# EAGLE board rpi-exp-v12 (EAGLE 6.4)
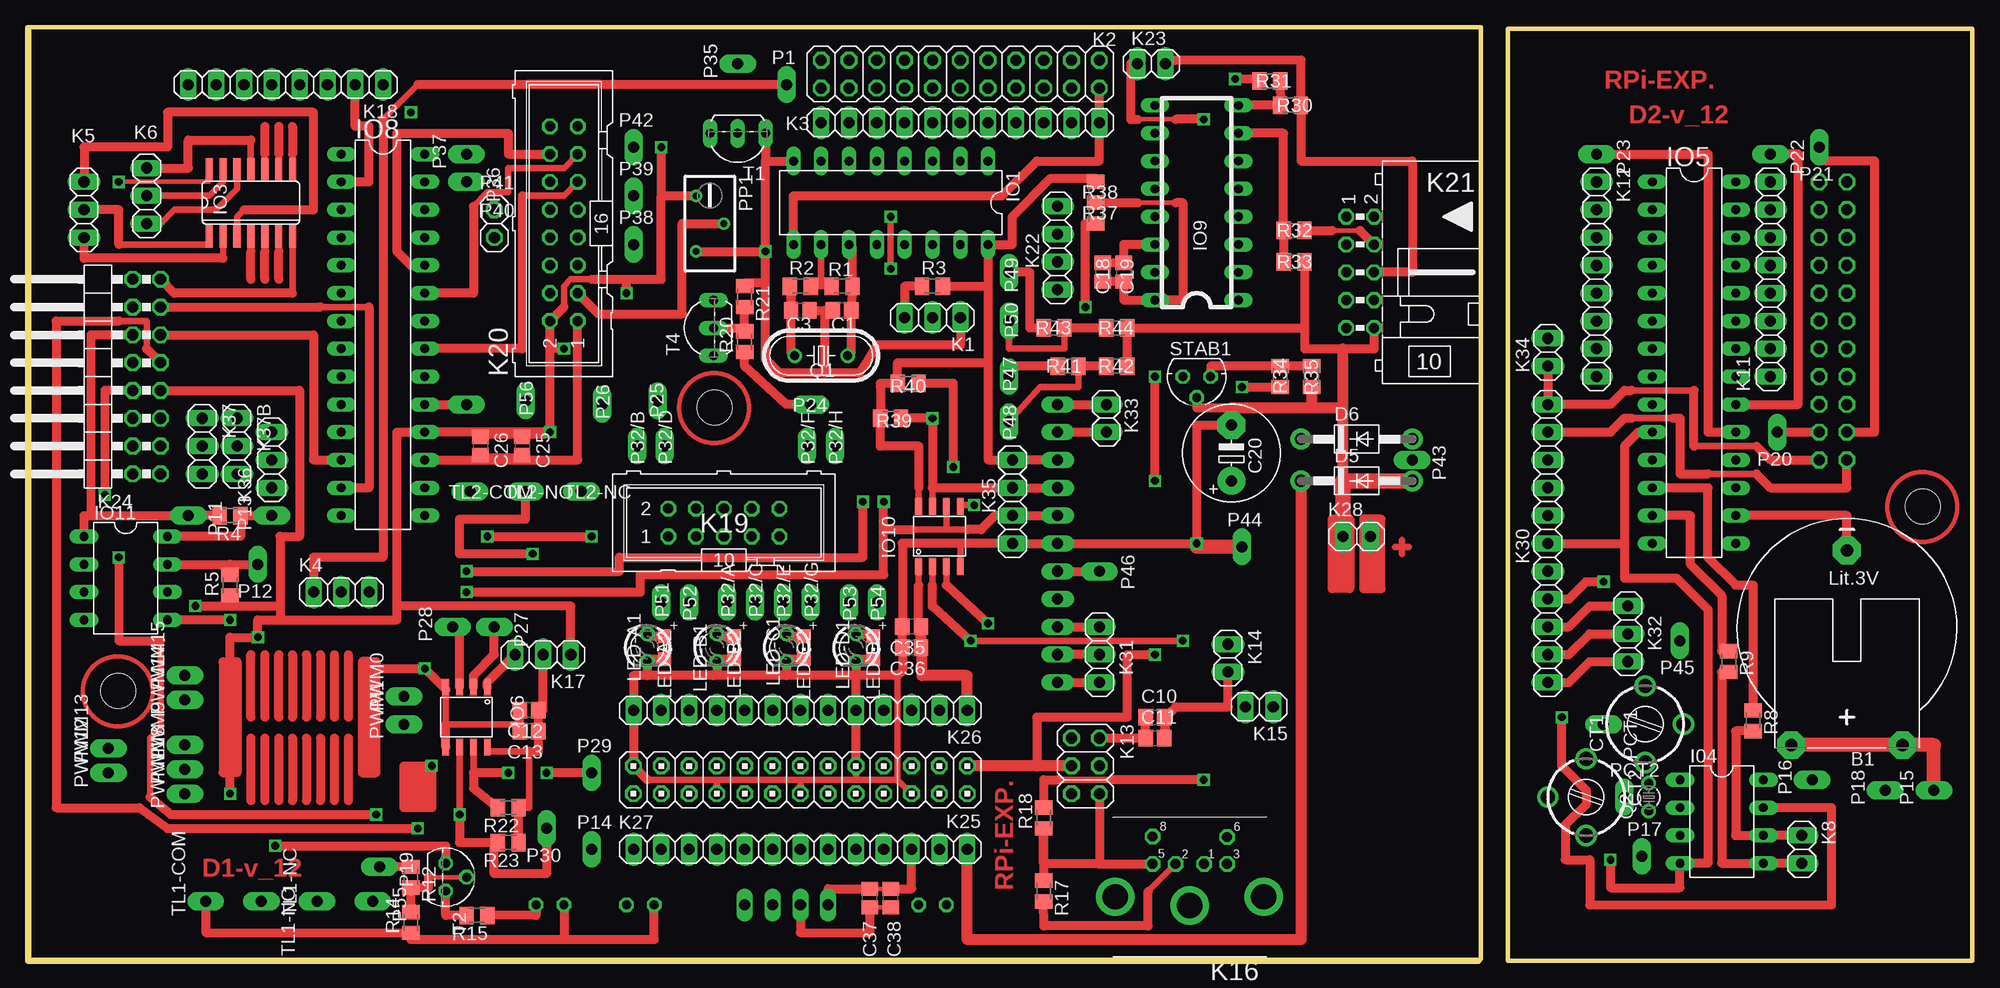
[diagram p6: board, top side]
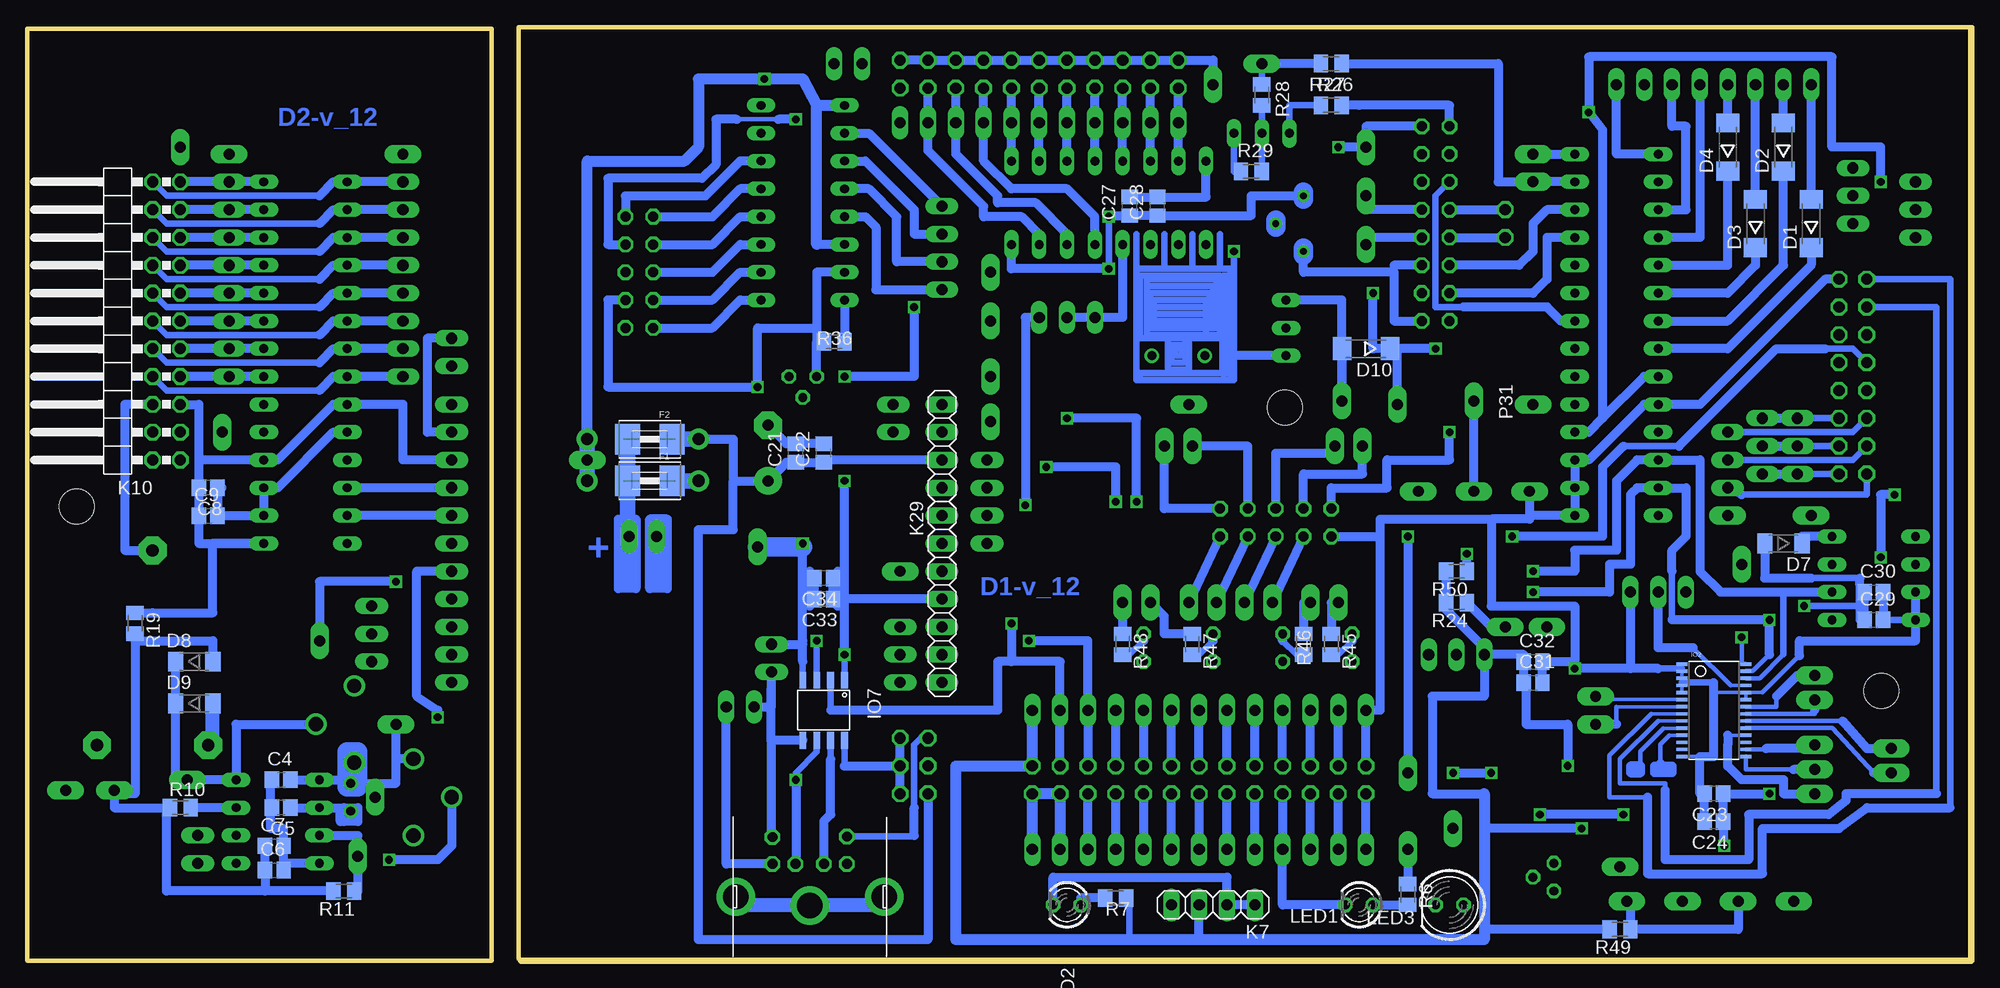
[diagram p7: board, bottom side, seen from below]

Size 177.57 x 85.23 mm. Coordinates in mm from the lower left corner, seen from the top.
Outline: 132.7,0.15 132.7,85.23 0,85.23 0,0.47
Outline: 132.49,0 0.09,0 0.09,85.09
Outline: 135.18,85.09 177.57,85.09 177.57,0 135.18,0 135.18,85.09
Copper layers (1*16): Top 0.035mm / dielectric 1.5mm / Bottom 0.035mm
Design rules "default": minimum track width 10mil, minimum drill 24mil, track to track 8mil, track to pad 8mil, pad to pad 8mil, via to via 8mil, smd to smd 8mil, copper to edge 40mil, drill to drill 8mil, minimum pad ring 10mil, minimum via ring 8mil, stop-mask expansion 4mil, vias tented up to drill 0mil, thermal gap 10mil
Holes 3.2 mm at 62.76,50.5 8.3,24.63 173.08,41.46

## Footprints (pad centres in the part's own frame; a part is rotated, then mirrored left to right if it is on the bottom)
CR2032H = drill 1.118 pad 2.54 octagon: + 5.08,10.795; +@1 -5.08,10.795; - 0,-6.985
0805 = smd 1.3 x 1.5: 1 -0.85,0; 2 0.85,0
E5-8,5 = drill 1.016 pad 2.54: + -2.54,0 | drill 1.016 pad 2.54 octagon: - 2.54,0
CTRIM3040.427 = drill 1.3: 1A -3.5,0; 1B 3.5,0; 2 0,-3.5
SOD106A-R = smd 1.7 x 2.1: A 2.2,0; C -2.2,0
DO41-10 = drill 1.118 pad 1.93: A 5.08,0; C -5.08,0
SOD80 = smd 1.4 x 1.8: 1 -1.7,0; 2 1.7,0
1812 = smd 2.286 x 2.794: 1 -2.046,0; 2 2.046,0
DIL08 = drill 0.813 long: 1 -3.81,-3.81; 2 -1.27,-3.81; 3 1.27,-3.81; 4 3.81,-3.81; 5 3.81,3.81; 6 1.27,3.81; 7 -1.27,3.81; 8 -3.81,3.81
DIL16 = drill 0.813 long: 1 -8.89,-3.81; 2 -6.35,-3.81; 3 -3.81,-3.81; 4 -1.27,-3.81; 5 1.27,-3.81; 6 3.81,-3.81; 7 6.35,-3.81; 8 8.89,-3.81; 9 8.89,3.81; 10 6.35,3.81; 11 3.81,3.81; 12 1.27,3.81; 13 -1.27,3.81; 14 -3.81,3.81; 15 -6.35,3.81; 16 -8.89,3.81
TSSOP28 = smd 0.305 x 0.991: 1 -4.225,-2.918; 2 -3.575,-2.918; 3 -2.925,-2.918; 4 -2.275,-2.918; 5 -1.625,-2.918; 6 -0.975,-2.918; 7 -0.325,-2.918; 8 0.325,-2.918; 9 0.975,-2.918; 10 1.625,-2.918; 11 2.275,-2.918; 12 2.925,-2.918; 13 3.575,-2.918; 14 4.225,-2.918; 15 4.225,2.918; 16 3.575,2.918; 17 2.925,2.918; 18 2.275,2.918; 19 1.625,2.918; 20 0.975,2.918; 21 0.325,2.918; 22 -0.325,2.918; 23 -0.975,2.918; 24 -1.625,2.918; 25 -2.275,2.918; 26 -2.925,2.918; 27 -3.575,2.918; 28 -4.225,2.918
SO14 = smd 0.66 x 2.032: 1 -3.81,-3.073; 2 -2.54,-3.073; 3 -1.27,-3.073; 4 0,-3.073; 5 1.27,-3.073; 6 2.54,-3.073; 7 3.81,-3.073; 8 3.81,3.073; 9 2.54,3.073; 10 1.27,3.073; 11 0,3.073; 12 -1.27,3.073; 13 -2.54,3.073; 14 -3.81,3.073
DIL28-3 = drill 0.813 long: 1 -16.51,-3.81; 2 -13.97,-3.81; 3 -11.43,-3.81; 4 -8.89,-3.81; 5 -6.35,-3.81; 6 -3.81,-3.81; 7 -1.27,-3.81; 8 1.27,-3.81; 9 3.81,-3.81; 10 6.35,-3.81; 11 8.89,-3.81; 12 11.43,-3.81; 13 13.97,-3.81; 14 16.51,-3.81; 15 16.51,3.81; 16 13.97,3.81; 17 11.43,3.81; 18 8.89,3.81; 19 6.35,3.81; 20 3.81,3.81; 21 1.27,3.81; 22 -1.27,3.81; 23 -3.81,3.81; 24 -6.35,3.81; 25 -8.89,3.81; 26 -11.43,3.81; 27 -13.97,3.81; 28 -16.51,3.81
SO8-COOL = smd 0.61 x 1.524: 1 -1.905,-2.743; 2 -0.635,-2.743; 3 0.635,-2.743; 4 1.905,-2.743; 5 1.905,2.743; 6 0.635,2.743; 7 -0.635,2.743; 8 -1.905,2.743
DIP16 = drill 0.8 long: P$1 -10.16,-3.81; P$2 -7.62,-3.81; P$3 -5.08,-3.81; P$4 -2.54,-3.81; P$5 0,-3.81; P$6 2.54,-3.81; P$7 5.08,-3.81; P$8 7.62,-3.81; P$9 7.62,3.81; P$10 5.08,3.81; P$11 2.54,3.81; P$12 0,3.81; P$13 -2.54,3.81; P$14 -5.08,3.81; P$15 -7.62,3.81; P$16 -10.16,3.81
1X03 = drill 1.016 long: 1 -2.54,0; 2 0,0; 3 2.54,0
2X11 = drill 1.016 octagon: 1 -12.7,-1.27; 2 -12.7,1.27; 3 -10.16,-1.27; 4 -10.16,1.27; 5 -7.62,-1.27; 6 -7.62,1.27; 7 -5.08,-1.27; 8 -5.08,1.27; 9 -2.54,-1.27; 10 -2.54,1.27; 11 0,-1.27; 12 0,1.27; 13 2.54,-1.27; 14 2.54,1.27; 15 5.08,-1.27; 16 5.08,1.27; 17 7.62,-1.27; 18 7.62,1.27; 19 10.16,-1.27; 20 10.16,1.27; 21 12.7,-1.27; 22 12.7,1.27
1X11 = drill 1.016 long: 1 -12.7,0; 2 -10.16,0; 3 -7.62,0; 4 -5.08,0; 5 -2.54,0; 6 0,0; 7 2.54,0; 8 5.08,0; 9 7.62,0; 10 10.16,0; 11 12.7,0
1X04 = drill 1.016 long: 1 -3.81,0; 2 -1.27,0; 3 1.27,0; 4 3.81,0
1X02 = drill 1.016 long: 1 -1.27,0; 2 1.27,0
2X11/90 = drill 1.016 octagon: 1 -12.7,-6.35; 2 -12.7,-3.81; 3 -10.16,-6.35; 4 -10.16,-3.81; 5 -7.62,-6.35; 6 -7.62,-3.81; 7 -5.08,-6.35; 8 -5.08,-3.81; 9 -2.54,-6.35; 10 -2.54,-3.81; 11 0,-6.35; 12 0,-3.81; 13 2.54,-6.35; 14 2.54,-3.81; 15 5.08,-6.35; 16 5.08,-3.81; 17 7.62,-6.35; 18 7.62,-3.81; 19 10.16,-6.35; 20 10.16,-3.81; 21 12.7,-6.35; 22 12.7,-3.81
1X08 = drill 1.016 long: 1 -8.89,0; 2 -6.35,0; 3 -3.81,0; 4 -1.27,0; 5 1.27,0; 6 3.81,0; 7 6.35,0; 8 8.89,0
2X03 = drill 1.016 octagon: 1 -2.54,-1.27; 2 -2.54,1.27; 3 0,-1.27; 4 0,1.27; 5 2.54,-1.27; 6 2.54,1.27
M_DIN6 = drill 0.9 pad 1.422 octagon: 1 -1.3,-3.75; 2 1.3,-3.75; 3 -3.4,-3.75; 5 3.4,-3.75; 6 -3.4,-6.2; 8 3.4,-6.25 | drill 2.3 pad 3.5: SH1 6.8,-0.75; SH2 0,0.05; SH3 -6.75,-0.75
ML10 = drill 0.914 octagon: 1 -5.08,-1.27; 2 -5.08,1.27; 3 -2.54,-1.27; 4 -2.54,1.27; 5 0,-1.27; 6 0,1.27; 7 2.54,-1.27; 8 2.54,1.27; 9 5.08,-1.27; 10 5.08,1.27
ML16 = drill 0.914 octagon: 1 -8.89,-1.27; 2 -8.89,1.27; 3 -6.35,-1.27; 4 -6.35,1.27; 5 -3.81,-1.27; 6 -3.81,1.27; 7 -1.27,-1.27; 8 -1.27,1.27; 9 1.27,-1.27; 10 1.27,1.27; 11 3.81,-1.27; 12 3.81,1.27; 13 6.35,-1.27; 14 6.35,1.27; 15 8.89,-1.27; 16 8.89,1.27
ML10L = drill 0.914 octagon: 1 -5.08,-1.27; 2 -5.08,1.27; 3 -2.54,-1.27; 4 -2.54,1.27; 5 0,-1.27; 6 0,1.27; 7 2.54,-1.27; 8 2.54,1.27; 9 5.08,-1.27; 10 5.08,1.27
2X08/90 = drill 1.016 octagon: 1 -8.89,-6.35; 2 -8.89,-3.81; 3 -6.35,-6.35; 4 -6.35,-3.81; 5 -3.81,-6.35; 6 -3.81,-3.81; 7 -1.27,-6.35; 8 -1.27,-3.81; 9 1.27,-6.35; 10 1.27,-3.81; 11 3.81,-6.35; 12 3.81,-3.81; 13 6.35,-6.35; 14 6.35,-3.81; 15 8.89,-6.35; 16 8.89,-3.81
2X13 = drill 1.016 octagon: 1 -15.24,-1.27; 2 -15.24,1.27; 3 -12.7,-1.27; 4 -12.7,1.27; 5 -10.16,-1.27; 6 -10.16,1.27; 7 -7.62,-1.27; 8 -7.62,1.27; 9 -5.08,-1.27; 10 -5.08,1.27; 11 -2.54,-1.27; 12 -2.54,1.27; 13 0,-1.27; 14 0,1.27; 15 2.54,-1.27; 16 2.54,1.27; 17 5.08,-1.27; 18 5.08,1.27; 19 7.62,-1.27; 20 7.62,1.27; 21 10.16,-1.27; 22 10.16,1.27; 23 12.7,-1.27; 24 12.7,1.27; 25 15.24,-1.27; 26 15.24,1.27
1X13 = drill 1.016 long: 1 -15.24,0; 2 -12.7,0; 3 -10.16,0; 4 -7.62,0; 5 -5.08,0; 6 -2.54,0; 7 0,0; 8 2.54,0; 9 5.08,0; 10 7.62,0; 11 10.16,0; 12 12.7,0; 13 15.24,0
LED3MM = drill 0.813 octagon: A -1.27,0; K 1.27,0
LED5MM = drill 0.813 octagon: A -1.27,0; K 1.27,0
CHIP-LED0805 = smd 1.2 x 1.2: A 0,-1.05; C 0,1.05
1X01_OVAL = drill 1 pad 1.676 long: 1 0,0
1X01 = drill 1.016 octagon: 1 0,0
RTRIM3296Y = drill 0.61: 1 1.27,-2.54; 2 -1.27,0; 3 1.27,2.54
HC49U-V = drill 0.813: 1 -2.413,0; 2 2.413,0
TC26V = drill 0.813: 1 -1.27,0; 2 1.27,0
M0805 = smd 1.3 x 1.6: 1 -0.95,0; 2 0.95,0
TO92 = drill 0.813 octagon: 1 -1.27,0; 2 0,1.905; 3 1.27,0
TO92-EBC-OVAL = drill 0.813 long: B 0,-1.27; C 2.54,-1.27; E -2.54,-1.27
TO92' = drill 0.813 octagon: 1 1.27,0; 2 0,1.905; 3 -1.27,0

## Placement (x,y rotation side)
B1  CR2032H  [CR2032H]  166.14,30.48 180 top
C1  22p - 37p  [0805]  74.39,59.37 180 top
C3  100p  [0805]  70.58,59.37 0 top
C4  *1  [0805]  154.4,16.51 0 bottom
C5  *1  [0805]  154.4,13.97 180 bottom
C6  100p  [0805]  155.03,8.25 0 bottom
C7  100n  [0805]  155.03,10.48 0 bottom
C8  100n  [0805]  161.06,43.18 180 bottom
C9  100p  [0805]  161.06,40.64 0 bottom
C10  100n  [0805]  102.96,22.22 0 top
C11  100p  [0805]  102.96,20.32 0 top
C12  100n  [0805]  45.81,22.86 180 top
C13  100p  [0805]  45.81,20.96 180 top
C18  100n  [0805]  98.2,62.86 270 top
C19  100p  [0805]  100.1,62.86 270 top
C20  470u / 10V  [E5-8,5]  109.95,46.36 90 top
C21  100n  [0805]  107.41,46.36 90 bottom
C22  100p  [0805]  104.87,46.36 90 bottom
C23  100n  [0805]  23.59,15.24 180 bottom
C24  100p  [0805]  23.59,12.7 180 bottom
C25  100n  [0805]  45.18,46.99 270 top
C26  100p  [0805]  41.37,46.99 270 top
C27  100n  [0805]  76.93,68.9 90 bottom
C28  100p  [0805]  74.39,68.9 90 bottom
C29  100p  [0805]  8.98,31.11 0 bottom
C30  100n  [0805]  8.98,33.66 0 bottom
C31  100p  [0805]  40.1,25.4 0 bottom
C32  100n  [0805]  40.1,27.31 0 bottom
C33  100p  [0805]  104.87,33.02 180 bottom
C34  100n  [0805]  104.87,34.92 180 bottom
C35  100p  [0805]  80.74,30.48 180 top
C36  100n  [0805]  80.74,28.57 180 top
C37  100p  [0805]  76.93,5.72 90 top
C38  100n  [0805]  78.83,5.72 90 top
CT1  [CTRIM3040.427]  147.73,21.59 90 top
CT2  [CTRIM3040.427]  142.33,14.92 270 top
D1  1N4148  [SOD106A-R]  14.7,67.31 90 bottom
D2  1N4148  [SOD106A-R]  17.24,74.3 90 bottom
D3  1N4148  [SOD106A-R]  19.78,67.31 90 bottom
D4  1N4148  [SOD106A-R]  22.32,74.3 90 bottom
D5  P6KE6V8A  [DO41-10]  121.38,43.81 0 top
D6  P6KE6V8A  [DO41-10]  121.38,47.62 0 top
D7  1N4148  [SOD80]  17.24,38.1 180 bottom
D8  1N4148  [SOD80]  162.33,27.31 0 bottom
D9  1N4148  [SOD80]  162.33,23.5 0 bottom
D10  1N4148  [SOD106A-R]  55.34,55.88 180 bottom
F1  [1812]  120.74,43.81 180 bottom
F2  [1812]  120.74,47.62 180 bottom
I04  PCF8583P  [DIL08]  154.71,12.7 270 top
IO1  4060N  [DIL16]  78.83,69.22 180 top
IO2  [TSSOP28]  23.59,22.86 270 bottom
IO3  4011D  [SO14]  20.41,69.22 0 top
IO5  MCP23017SP  [DIL28-3]  152.17,54.61 270 top
IO6  ADUM1250  [SO8-COOL]  40.1,22.22 180 top
IO7  ADUM1250  [SO8-COOL]  104.87,22.86 180 bottom
IO8  MCP23017SP  [DIL28-3]  32.48,57.15 270 top
IO9  MCP3208  [DIP16]  106.77,70.48 90 top
IO10  TCA9517 / ISO1540 / ADuM1250  [SO8-COOL]  83.28,38.73 0 top
IO11  PCF8583P  [DIL08]  8.98,34.92 270 top
K1  [1X03]  82.64,58.74 180 top
K2  [2X11]  85.18,80.96 0 top
K3  [1X11]  85.18,76.52 0 top
K4  [1X03]  28.67,33.66 0 top
K5  [1X03]  5.17,68.58 270 top
K6  [1X03]  10.89,69.85 270 top
K7  [1X04]  69.31,5.08 180 bottom
K8  [1X02]  162.02,10.16 270 top
K10  [2X11/90]  169.95,58.42 90 bottom
K11  [1X08]  159.16,62.23 90 top
K12  [1X08]  143.28,62.23 270 top
K13  [2X03]  96.61,17.78 270 top
K14  [1X02]  109.63,27.62 270 top
K15  [1X02]  112.49,23.18 180 top
K16  [M_DIN6]  106.14,5.08 180 top
K17  [1X03]  47.08,27.94 180 top
K18  [1X08]  23.59,80.01 180 top
K19  [ML10]  63.59,40 0 top
K20  [ML16]  48.99,67.31 90 top
K21  [ML10L]  121.69,62.86 270 top
K22  [1X04]  94.07,65.09 90 top
K23  [1X02]  102.64,81.91 180 top
K24  [2X08/90]  5.81,53.34 90 top
K25  [2X13]  70.58,16.51 180 top
K26  [1X13]  70.58,22.86 180 top
K27  [1X13]  70.58,10.16 0 top
K28  [1X02]  121.38,38.73 0 top
K29  [1X11]  94.07,38.1 270 bottom
K30  [1X11]  138.84,38.1 270 top
K31  [1X03]  97.88,27.94 270 top
K32  [1X03]  146.14,29.84 270 top
K33  [1X02]  98.52,49.53 90 top
K34  [1X02]  138.84,55.56 270 top
K35  [1X04]  89.94,41.91 90 top
K36  [1X03]  22.32,45.72 90 top
K37  [1X03]  15.97,46.99 270 top
K37B  [1X03]  19.14,46.99 270 top
LED1  [LED3MM]  55.97,5.08 180 bottom
LED2  [LED3MM]  82.64,5.08 180 bottom
LED3  [LED5MM]  47.72,5.08 180 bottom
LED-A1  [LED3MM]  56.61,28.57 270 top
LED-A2  [CHIP-LED0805]  58.19,28.57 180 top
LED-B1  [LED3MM]  62.96,28.57 270 top
LED-B2  [CHIP-LED0805]  64.54,28.57 180 top
LED-C1  [LED3MM]  69.31,28.57 270 top
LED-C2  [CHIP-LED0805]  70.89,28.57 180 top
LED-D1  [LED3MM]  75.66,28.57 270 top
LED-D2  [CHIP-LED0805]  77.24,28.57 180 top
P1  [1X01_OVAL]  69.31,80.01 0 top
P11  [1X01_OVAL]  14.7,40.64 270 top
P12  [1X01_OVAL]  21.05,36.19 180 top
P13  [1X01_OVAL]  22.32,40.64 90 top
P14  [1X01_OVAL]  51.53,10.16 0 top
P15  [1X01_OVAL]  174.08,15.56 90 top
P16  [1X01_OVAL]  162.97,16.51 90 top
P17  [1X01_OVAL]  147.41,9.53 0 top
P18  [1X01_OVAL]  169.64,15.56 90 top
P19  [1X01_OVAL]  32.16,8.57 270 top
P20  [1X01_OVAL]  159.79,48.26 180 top
P21  [1X01_OVAL]  163.6,74.3 180 top
P22  [1X01_OVAL]  159.16,73.66 270 top
P23  [1X01_OVAL]  143.28,73.66 270 top
P24  [1X01_OVAL]  71.53,50.8 90 top
P25  [1X01_OVAL]  57.56,51.12 180 top
P26  [1X01_OVAL]  52.48,50.8 0 top
P27  [1X01_OVAL]  42.64,30.48 270 top
P28  [1X01_OVAL]  38.83,30.48 90 top
P29  [1X01_OVAL]  51.53,17.15 0 top
P30  [1X01_OVAL]  47.4,12.06 180 top
P31  [1X01_OVAL]  40.1,50.8 90 bottom
P32/A  [1X01_OVAL]  63.91,32.7 0 top
P32/B  [1X01_OVAL]  55.65,46.99 0 top
P32/C  [1X01_OVAL]  66.45,32.7 0 top
P32/D  [1X01_OVAL]  58.19,46.99 0 top
P32/E  [1X01_OVAL]  68.99,32.7 0 top
P32/F  [1X01_OVAL]  71.21,46.99 0 top
P32/G  [1X01_OVAL]  71.53,32.7 0 top
P32/H  [1X01_OVAL]  73.75,46.99 0 top
P35  [1X01_OVAL]  64.86,81.91 90 top
P36  [1X01_OVAL]  40.1,71.12 270 top
P37  [1X01_OVAL]  40.1,73.66 90 top
P38  [1X01_OVAL]  55.34,65.41 0 top
P39  [1X01_OVAL]  55.34,69.85 0 top
P40  [1X01]  42.64,66.04 0 top
P41  [1X01]  42.64,68.58 0 top
P42  [1X01_OVAL]  55.34,74.3 0 top
P43  [1X01_OVAL]  126.46,45.72 270 top
P44  [1X01_OVAL]  110.9,37.78 0 top
P45  [1X01_OVAL]  150.9,29.21 180 top
P46  [1X01_OVAL]  97.88,35.56 90 top
P47  [1X01_OVAL]  89.63,53.34 180 top
P48  [1X01_OVAL]  89.63,49.21 0 top
P49  [1X01_OVAL]  89.63,62.86 180 top
P50  [1X01_OVAL]  89.63,58.42 180 top
P51  [1X01_OVAL]  57.88,32.7 0 top
P52  [1X01_OVAL]  60.42,32.7 0 top
P53  [1X01_OVAL]  75.02,32.7 0 top
P54  [1X01_OVAL]  77.56,32.7 0 top
P55  [1X01_OVAL]  31.52,5.4 270 top
P56  [1X01_OVAL]  45.49,51.12 180 top
PCT1  [1X01_OVAL]  143.92,21.59 270 top
PCT2  [1X01_OVAL]  145.82,14.92 0 top
PP1  [RTRIM3296Y]  62.32,67.31 180 top
PWM0  [1X01_OVAL]  34.38,24.13 90 top
PWM1  [1X01_OVAL]  34.38,21.59 90 top
PWM8  [1X01_OVAL]  14.38,17.46 90 top
PWM9  [1X01_OVAL]  14.38,19.69 90 top
PWM11  [1X01_OVAL]  14.38,15.24 90 top
PWM12  [1X01_OVAL]  7.39,17.15 90 top
PWM13  [1X01_OVAL]  7.39,19.37 90 top
PWM14  [1X01_OVAL]  14.38,23.81 90 top
PWM15  [1X01_OVAL]  14.38,26.03 90 top
Q1  4.000MHz  [HC49U-V]  72.48,55.25 180 top
Q2  [TC26V]  148.05,14.92 90 top
R1  470k  [M0805]  74.39,61.59 180 top
R2  2k2  [M0805]  70.58,61.59 0 top
R3  56k  [M0805]  82.64,61.59 0 top
R4  56k  [M0805]  18.51,40.64 180 top
R5  56k  [M0805]  18.51,34.29 90 top
R6  1k5  [M0805]  51.53,6.03 270 bottom
R7  1k  [M0805]  78.2,5.72 180 bottom
R8  *2  [M0805]  157.57,21.91 270 top
R9  *2  [M0805]  155.35,27.31 270 top
R10  56k  [M0805]  163.6,13.97 0 bottom
R11  *3  [M0805]  148.68,6.35 180 bottom
R12  3k3  [M0805]  35.02,7.62 270 top
R14  56k  [M0805]  35.02,3.49 90 top
R15  1k  [M0805]  41.05,4.13 180 top
R17  56k  [M0805]  92.8,6.35 270 top
R18  56k  [M0805]  92.8,13.02 90 top
R19  *4  [M0805]  167.73,30.8 270 bottom
R20  1k  [M0805]  65.5,56.52 90 top
R21  ----  [M0805]  65.5,60.64 270 top
R22  56k  [M0805]  43.91,13.97 180 top
R23  56k  [M0805]  43.91,10.79 180 top
R24  ----  [M0805]  47.08,32.7 180 bottom
R26  [M0805]  58.51,78.11 0 bottom
R27  [M0805]  58.51,81.91 180 bottom
R28  [M0805]  64.86,79.06 270 bottom
R29  [M0805]  65.81,72.07 0 bottom
R30  [M0805]  115.34,78.11 0 top
R31  [M0805]  113.44,80.33 0 top
R32  [M0805]  115.66,66.67 0 top
R33  [M0805]  115.66,63.82 180 top
R34  [M0805]  114.39,53.34 270 top
R35  [M0805]  117.25,53.34 90 top
R36  [M0805]  103.91,56.52 0 bottom
R37  [M0805]  97.56,68.26 270 top
R38  [M0805]  97.56,70.17 90 top
R39  56k  [M0805]  78.83,49.53 0 top
R40  56k  [M0805]  80.42,52.7 0 top
R41  10k  [M0805]  95.02,54.29 180 top
R42  18k  [M0805]  99.47,54.29 180 top
R43  10k  [M0805]  93.75,57.78 180 top
R44  18k  [M0805]  99.47,57.78 180 top
R45  1k5  [M0805]  58.51,28.89 270 bottom
R46  1k5  [M0805]  61.05,28.89 270 bottom
R47  1k5  [M0805]  71.21,28.89 270 bottom
R48  1k5  [M0805]  77.56,28.89 270 bottom
R49  (56k)  [M0805]  32.16,2.86 180 bottom
R50  (56k)  [M0805]  47.08,35.56 180 bottom
STAB1  TL431  [TO92]  106.77,53.34 180 top
T1  (NPN)  [TO92-EBC-OVAL]  64.86,74.3 180 top
T2  (PNP)  [TO92']  38.19,7.62 270 top
T4  (NPN)  [TO92-EBC-OVAL]  61.37,57.78 90 top
TL1-COM  [1X01_OVAL]  16.28,5.4 90 top
TL1-NC  [1X01_OVAL]  26.44,5.4 90 top
TL1-NO  [1X01_OVAL]  21.36,5.4 270 top
TL2-COM  [1X01_OVAL]  40.41,42.86 90 top
TL2-NC  [1X01_OVAL]  50.57,42.86 90 top
TL2-NO  [1X01_OVAL]  45.49,42.86 90 top

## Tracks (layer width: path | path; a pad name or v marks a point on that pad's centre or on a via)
5VRPI
  Top 1.016: D5.C 116.3,1.91 85.82,1.91 K27.13
  Bottom 1.016: K27.13 K25.2 K25.4 K27.12
  Bottom 1.422: D5.C F1.1
4011-4
  Top 0.61: IO3.4 20.41,64.77
  Top 0.813: 20.41,62.23 20.41,64.77
4011-5
  Top 0.61: IO3.5 21.68,64.77
  Top 0.813: 21.68,62.23 21.68,64.77
4011-6
  Top 0.61: IO3.6 22.95,64.77
  Top 0.813: 22.95,62.23 22.95,64.77
4011-8
  Top 0.61: IO3.8 24.22,73.66
  Top 0.813: 24.22,76.2 24.22,73.66
4011-9
  Top 0.61: IO3.9 22.95,73.66
  Top 0.813: 22.95,76.2 22.95,73.66
4011-10
  Top 0.61: IO3.10 21.68,73.66
  Top 0.813: 21.68,76.2 21.68,73.66
+3V  (via drill 0.7)
  Top 0.305: 82.01,30.48 C35.1
  Top 0.406: C38.1 C37.1
  Top 0.61: 10.89,55.88 10.89,58.42 8.35,58.42 | IO10.1 81.37,34.29 | 81.37,31.11 81.37,30.48 C35.1
  Top 0.813: v102.96,43.81 v102.96,53.34 | v102.96,27.94 100.42,27.94 100.42,22.22 92.17,22.22 92.17,17.78 | IO6.1 42,25.4 K17.3 | v35.65,12.06 12.79,12.06 10.25,13.97 2.63,13.97 2.63,58.42 8.35,58.42 | K24.9 10.89,55.88 | C37.1 76.93,2.54 70.58,2.54 K7.3 | v36.92,17.78 36.92,13.97 34.38,13.97 34.38,17.78 v36.92,17.78 | v36.92,17.78 36.29,17.78 36.29,14.6 35.02,14.6 35.02,17.15 35.65,17.15 35.65,15.24 | 81.37,31.11 81.37,34.29 | v96.61,59.69 96.61,67.31 R37.2
  Top 1.016: K13.3 92.17,17.78 K25.1 | C35.1 C36.1 81.69,28.57 81.69,26.03 85.82,26.03 K26.1
  Bottom 0.305: 102.96,31.75 102.96,33.02 | 102.96,33.34 102.96,34.92 v102.96,43.81 | C32.1 40.95,27.94 | 44.54,12.06 44.54,15.24
  Bottom 0.406: C34.1 104.23,34.92 | 102.96,31.75 v102.96,27.94 | R7.1 76.93,5.72
  Bottom 0.61: 102.96,34.92 C34.1 | 76.93,5.72 76.93,1.91 | 40.73,25.19 C31.1 | IO7.1 v102.96,27.94
  Bottom 0.813: C34.1 C33.1 103.6,33.02 | v102.96,27.94 102.96,33.02 | v102.96,43.81 102.96,33.34 102.96,33.02 | C31.1 C32.1 | 40.95,27.94 K17.3 | v35.65,12.06 44.54,12.06 | 44.54,15.24 49.3,15.24 49.3,24.13 44.54,24.13 K17.3 | 40.73,25.19 40.73,21.59 36.92,21.59 v36.92,17.78 | 103.6,32.39 103.6,33.02 | 103.6,33.02 103.6,35.56 | K17.3 44.54,28.57 48.03,32.07 R24.2 R50.2 | R49.2 44.54,2.86 44.54,2.22 | v96.61,59.69 96.61,53.34 v102.96,53.34 | K29.8 102.96,33.02 | 76.93,1.91 70.58,1.91 K7.3
  Bottom 1.016: K26.1 K25.1 92.8,17.78 92.8,1.91 76.93,1.91 44.54,1.91 44.54,2.22 44.54,15.24
+3VB2  (via drill 0.7)
  Top 0.813: v143.92,34.61 142.33,34.61 140.74,33.02 K30.8
  Bottom 0.813: v143.92,34.61 150.9,34.61 P45.1
+5V  (via drill 0.7)
  Top 0.406: C26.1 C25.1 47.3,47.84 v47.72,48.26 | IO3.14 16.6,71.12 v8.35,71.12
  Top 0.61: 48.99,59.69 48.99,61.59 49.62,62.23 51.53,62.23 | v78.83,63.18 v78.83,67.94 | IO10.8 81.37,43.18
  Top 0.813: v18.51,15.24 18.51,17.15 | 18.51,27.31 18.51,29.53 v21.05,29.53 21.05,31.11 23.08,31.11 | 23.08,31.11 33.75,31.11 33.75,32.39 | 33.75,32.39 33.75,48.26 IO8.18 v47.72,48.26 47.72,55.88 | 23.08,32.39 23.08,38.73 24.86,38.73 24.86,52.07 K24.7 | 23.08,32.39 23.08,31.11 | K17.1 49.62,32.39 33.75,32.39 | 87.72,61.59 IO1.16 89.94,65.41 89.94,67.94 93.44,71.44 97.56,71.44 R38.2 | 87.72,61.59 87.72,54.61 | 87.72,54.61 87.72,45.72 K35.4 K29.3 | 57.88,69.85 PP1.1 | 47.72,55.88 K20.2 48.99,59.69 | 57.88,69.85 57.88,62.23 54.7,62.23 | 18.51,17.15 19.14,17.15 19.14,27.31 18.51,27.31 | 18.51,17.15 18.51,27.31 | v15.33,32.39 18.51,32.39 | 18.51,32.39 23.08,32.39 | 51.53,62.23 54.7,62.23 | v48.99,55.88 47.72,55.88 | v54.7,60.96 54.7,62.23 | 87.72,54.61 79.47,54.61 R40.1 77.88,52.7 77.88,52.39 R39.1 77.88,46.99 81.37,46.99 81.37,43.18 | R3.2 87.72,61.59 | R5.1 18.51,32.39 | 17.87,27.31 17.87,17.15 18.51,17.15 | v22.63,10.48 38.19,10.48 T2.3 | v57.88,74.3 57.88,69.85
  Bottom 0.406: C30.1 10.25,33.66 | IO2.28 21.05,27.09 v21.05,29.53 | C29.1 9.83,32.39
  Bottom 0.61: 10.25,33.66 10.25,34.29 | v78.83,67.94 v78.83,63.18 | 10.25,34.92 14.7,34.92 | 9.83,32.39 v15.33,32.39
  Bottom 0.813: v18.51,15.24 C23.1 C24.1 22.74,10.48 v22.63,10.48 | C29.1 C30.1 | D6.C 113.12,47.62 113.12,43.81 | 113.12,43.81 C20.+ 108.26,45.5 C21.1 C22.1 104.87,45.72 K29.3 | K13.5 95.34,1.91 116.3,1.91 116.3,39.37 113.12,39.37 113.12,43.81 | v78.83,63.18 87.72,63.18 IO1.16 | v47.72,48.26 47.72,45.72 53.43,45.72 53.43,43.18 58.51,43.18 K19.2 | IO8.9 29.94,53.34 33.75,49.53 | 33.75,49.53 35.02,48.26 IO8.18 | 10.25,34.92 10.25,34.29 10.25,31.11 | v48.99,55.88 D10.C | D10.C 54.7,55.88 v54.7,60.96 | D7.2 18.94,34.92 14.7,34.92 | v78.83,67.94 78.73,68.05 C27.1 C28.1 65.81,68.05 65.81,69.85 PP1.1 | v8.35,71.12 8.35,74.3 12.79,74.3 12.79,82.55 35.02,82.55 v35.02,77.47 33.75,75.88 33.75,49.53 | P26.1 52.48,55.88 D10.C | K20.15 55.34,76.2 P42.1 v57.88,74.3
  Bottom 1.422: D6.C F2.1
  Bottom 1.778: 61.05,69.53 PP1.1 61.05,70.17
+5VB2
  Bottom 0.406: IO5.18 154.71,45.72 | 149.63,50.8 IO5.9 | 160.63,31.75 160.64,31.75
  Bottom 0.61: 147.09,50.8 IO5.9
  Bottom 0.813: IO5.18 161.91,45.72 | 161.91,45.72 C8.2 C9.1 161.91,38.1 IO5.15 160.64,38.1 160.64,31.75 166.14,31.75 166.46,31.75 R19.1 | 154.71,45.72 149.63,50.8 | K10.5 161.91,50.8 161.91,45.72 | 147.09,50.8 143.28,50.8 143.28,45.72 K30.3
AD-VCC
  Top 0.406: R38.1 105.5,69.21
  Top 0.813: R38.1 101.37,69.22 | C18.2 C19.2 100.1,60.33 IO9.P$16 105.5,60.33 105.5,69.21 105.5,69.22 104.87,69.22
  Bottom 0.813: IO9.P$16 R36.2
ADC0
  Bottom 0.813: K21.9 115.03,57.78 112.49,60.33 IO9.P$1
ADC1
  Bottom 0.813: K21.7 115.03,60.33 112.49,62.86 IO9.P$2
ADC2
  Bottom 0.813: K21.5 115.03,62.86 112.49,65.41 IO9.P$3
ADC3
  Bottom 0.813: K21.3 115.03,65.41 112.49,67.94 IO9.P$4
ADC4
  Bottom 0.813: IO9.P$5 112.49,70.48 115.03,67.94 K21.1
ADC5
  Bottom 0.813: K21.2 122.96,69.85 115.66,69.85 112.49,73.03 IO9.P$6
ADC6
  Top 0.813: R33.2 R32.1 114.71,75.56 IO9.P$7
ADC7
  Top 0.813: R31.2 R30.1 IO9.P$8
ADC-D6  (via drill 0.7)
  Top 0.406: 121.69,66.67 119.15,66.67 | 101.37,76.83 104.87,76.83
  Top 0.813: K21.4 121.69,66.67 | R32.2 119.15,66.67 | v107.41,76.83 104.87,76.83 | K23.2 100.74,81.91 100.74,76.83 101.37,76.83
  Bottom 0.406: 108.99,76.83 112.8,76.83
  Bottom 0.813: K21.4 124.55,65.41 124.55,71.44 115.98,71.44 114.71,72.71 114.71,76.83 112.8,76.83 | v107.41,76.83 108.99,76.83
ADC-D7
  Top 0.813: K21.6 126.46,62.86 126.46,73.03 116.29,73.03 R30.2 116.29,82.23 109.31,82.23 104.87,82.23 103.91,82.23 K23.1
BCKUP+
  Top 1.27: P15.1 174.08,19.69 B1.+
  Bottom 0.813: B1.+ 160.63,19.69
  Bottom 1.27: 160.63,19.69 D9.2
BCKUP-CNT
  Top 0.813: P13.1 R4.1 19.46,38.73 IO11.8
  Bottom 0.813: IO11.8 15.54,38.73 D7.1
CNT-IN
  Top 0.813: K24.12 5.81,57.15 5.81,40.64 | 5.81,40.64 5.17,40.64 IO11.1 | 5.81,40.64 P11.1 R4.2
CNT-INT
  Top 0.61: P12.1 19.27,36.19
  Top 0.813: IO11.7 18.51,36.19 | 18.51,36.19 P12.1 | R5.2 18.51,36.19
DIS-KONTR
  Top 0.813: K20.3 52.16,59.05 59.78,59.05 59.78,67.31 PP1.2
  Bottom 1.778: 63.59,67.63 PP1.2 63.59,66.99
FRQ0
  Bottom 0.813: IO1.7 K3.1 K2.1
FRQ1
  Bottom 0.813: IO1.5 K3.3 K2.5
FRQ2
  Bottom 0.813: IO1.4 K3.4 K2.7
FRQ3
  Bottom 0.813: IO1.6 K3.2 K2.3
FRQ4
  Bottom 0.813: K2.17 K3.9 92.8,73.66 88.99,69.85 88.99,69.22 85.5,69.22 82.64,66.36 IO1.14
FRQ5
  Bottom 0.813: K2.15 K3.8 90.26,73.03 87.72,70.48 82.64,70.48 80.1,67.94 IO1.13
FRQ6
  Bottom 0.813: K2.19 K3.10 95.34,73.98 90.26,68.9 90.26,67.94 86.77,67.94 85.18,66.36 IO1.15
FRQ7
  Bottom 0.813: IO1.1 K3.7 K2.13
FRQ8
  Bottom 0.813: IO1.2 K3.6 K2.11
FRQ9
  Bottom 0.813: IO1.3 K3.5 K2.9
FRQ10
  Top 0.813: IO1.9 69.94,69.85 88.99,69.85 92.17,73.03 97.88,73.03 K3.11 K2.21
G1  (via drill 0.7)
  Top 0.61: 40.73,17.15 IO6.7
  Top 0.813: R22.2 40.73,15.75 40.73,17.15 v43.91,17.15 | v42,38.73 v51.53,38.73 | P29.1 v47.4,17.15
  Bottom 0.61: K24.10 10.89,55.88 13.43,55.88 | 26.76,46.99 31.84,46.99
  Bottom 0.813: 26.76,46.99 17.87,55.88 13.43,55.88 | 31.84,46.99 33.75,45.08 33.75,38.73 v42,38.73 | v51.53,38.73 P29.1 | v47.4,17.15 v43.91,17.15
G2  (via drill 0.7)
  Top 0.61: 12.16,29.21 12.16,21.27 11.2,20.32 11.2,14.92 | v39.46,13.34 IO6.6
  Top 0.813: K24.8 7.08,52.07 v7.08,42.55 | v8.35,36.83 8.35,29.21 12.16,29.21 | 11.2,14.92 13.11,13.34 v31.84,13.34 | v39.46,13.34 39.46,10.79 R23.2 42.64,10.79 42.64,7.94 47.4,7.94 P30.1
  Bottom 0.813: v31.84,13.34 v39.46,13.34 | v7.08,42.55 8.35,42.55 v8.35,36.83
GND  (via drill 0.7)
  Top 0.305: 79.89,35.66 C35.2 | C25.2 41.79,46.14 41.37,45.72 | C13.2 44.96,21.59
  Top 0.406: C25.2 C26.2 | C38.2 C37.2
  Top 0.61: 79.47,26.03 79.47,16.51 | 79.47,16.51 K25.6 | 56.61,16.51 62.96,16.51 | 62.96,16.51 70.58,16.51 | 70.58,16.51 75.66,16.51 | 75.66,16.51 79.47,16.51 | K25.20 62.96,16.51 | K25.14 70.58,16.51 | K25.9 75.66,16.51 | IO3.7 24.22,60.96 | IO10.4 85.18,38.1 | 44.96,21.59 38.19,21.59 38.19,24.76 IO6.4 | v86.45,41.59 85.18,41.59 IO10.5
  Top 0.813: IO8.17 41.37,45.72 50.26,45.72 K20.1 | C20.- 106.77,48.89 v106.77,38.1 K29.6 K35.1 85.18,38.1 79.89,38.1 C35.2 C36.2 79.89,26.46 79.47,26.03 75.66,26.03 | 38.19,24.76 v36.29,26.67 31.84,26.67 | 72.8,59.37 C1.2 | 72.8,53.66 75.97,53.66 76.61,54.61 77.56,56.2 85.18,56.2 K1.1 | 72.8,53.66 68.67,53.66 67.4,54.93 67.4,61.91 | 67.4,61.91 v67.4,64.77 | PP1.3 v67.4,64.77 | T1.E 67.4,73.03 | 56.61,16.51 K25.25 K26.13 55.34,26.03 56.61,26.03 | v67.4,64.77 67.4,73.03 | 67.4,73.03 IO1.8 | K21.10 122.96,55.88 120.11,55.88 117.25,55.88 116.61,55.88 116.61,57.78 | 24.22,60.96 13.43,60.96 K24.15 | C38.2 80.74,6.56 K27.11 | 31.84,26.67 31.21,26.67 | 31.21,26.67 31.21,17.15 | 31.21,17.15 31.84,17.15 31.84,26.67 | 31.21,27.31 31.84,27.31 31.84,26.67 | 31.21,17.15 30.57,17.15 30.57,27.31 31.21,27.31 | 31.21,26.67 31.21,27.31 | 75.66,26.03 69.31,26.03 | 69.31,26.03 62.64,26.03 | 62.64,26.03 56.61,26.03 | K25.9 K26.5 75.66,26.03 | IO6.5 38.19,21.59 | C13.2 C12.2 | C3.2 72.8,59.37 | 72.8,59.37 72.8,53.66 | 75.66,26.03 LED-D1.K 75.88,27.53 LED-D2.C | 56.61,26.03 LED-A1.K 56.83,27.53 LED-A2.C | 62.64,26.03 62.96,26.35 LED-B1.K 63.18,27.53 LED-B2.C | 69.31,26.03 LED-C1.K 69.53,27.53 LED-C2.C | R21.1 65.5,61.91 67.4,61.91 | R31.1 112.49,80.52 v110.27,80.52 | R33.1 116.61,57.78 | 109.95,50.48 106.77,50.48 STAB1.2 | 48.99,1.91 57.24,1.91 LED1.K | 48.99,1.91 35.02,1.91 R14.1 16.28,2.54 TL1-COM.1 | K28.1 120.74,38.73 | 119.79,40 120.11,40 | 120.11,40 120.42,40 | 120.42,38.42 120.11,38.42 K28.1 | 119.15,38.73 K28.1 | 119.15,40.32 120.74,40.32 120.74,33.97 119.15,33.97 119.15,40.32 | 119.15,40.32 119.79,39.69 119.79,34.29 120.11,34.29 120.11,40
  Top 0.813: IO9.P$14 100.1,65.41 C19.1 C18.1 | 116.61,57.78 R44.1 R42.1 | K7.4 73.12,6.56 C37.2 | LED3.K 48.99,1.91
  Top 1.016: 120.11,40 120.11,50.48 | 120.11,50.48 117.25,50.48 | 117.25,50.48 109.95,50.48 C20.- | 106.77,37.78 v106.77,38.1 | R35.1 117.25,50.48 | 120.11,50.48 120.11,55.88
  Top 1.27: P44.1 106.77,37.78
  Top 1.422: D5.A 120.11,43.81 120.11,40 K28.1
  Bottom 0.305: IO2.14 24.86,18.63 | IO2.1 IO2.2 | IO2.2 IO2.3 26.5,25.4 IO2.4 IO2.5 | IO2.24 23.59,24.48 | IO2.24 IO2.23 | C23.2 24.86,15.24 | 36.29,27.31 v36.29,26.67 | 26.5,26.67 IO2.2 | IO2.24 19.14,24.48
  Bottom 0.406: 35.02,45.72 IO8.17 | 19.14,24.48 15.76,27.86 | 105.5,34.92 C34.2 106.77,34.92
  Bottom 0.61: IO8.10 29.94,50.8 | 23.59,25.4 26.5,25.4 | v36.29,26.67 31.21,26.67 28.67,26.67 26.5,26.67 | C29.2 IO11.4 | IO9.P$9 103.6,78.11 | 108.26,47.2 C21.2 | 106.77,25.4 IO7.4 | IO7.4 106.77,27.31 | 106.77,33.66 106.77,34.92 106.77,37.78 | 52.8,62.86 52.8,63.5 | IO7.4 106.77,29.21 | v67.4,64.77 67.4,53.02 76.29,53.02 76.29,63.18 | 76.29,66.36 76.29,63.18 | 76.29,63.18 73.75,63.18 | 73.75,66.36 73.75,63.18 | 73.75,63.18 71.21,63.18 | 71.21,66.36 71.21,63.18 | 71.21,63.18 68.67,63.18 | 68.67,66.36 68.67,63.18 | 68.67,63.18 67.72,63.18 67.72,62.55 | 67.72,62.55 67.72,53.02 75.97,53.02 75.97,53.66 68.35,53.66 68.04,53.66 68.04,55.25 68.04,62.55 | 68.04,62.55 67.72,62.55 | 69.94,56.83 68.35,56.83 68.35,62.55 68.04,62.55 | 71.53,56.83 71.85,56.83 | 73.43,56.83 75.97,56.83 75.97,62.55 68.67,62.55 68.67,57.15 75.34,57.15 75.34,57.78 | 75.34,61.59 75.34,62.23 68.99,62.23 68.99,57.78 75.34,57.78 | 75.34,57.78 75.34,61.59 | 75.34,61.59 69.31,61.59 69.31,58.1 75.02,58.1 75.02,60.96 69.62,60.96 69.62,58.42 74.7,58.42 74.7,59.05 | 74.7,59.69 74.7,60.33 69.94,60.33 69.94,59.69 | 69.94,59.69 69.94,59.05 | 69.94,59.05 74.7,59.05 | 74.7,59.05 74.7,59.69 | 74.7,59.69 69.94,59.69 | 69.94,59.05 69.94,56.83 | 69.94,56.83 71.53,56.83 | 71.53,56.83 71.53,53.97 73.43,53.97 73.43,56.83 | 73.43,56.83 71.85,56.83 | 71.85,56.83 71.85,54.61 73.12,54.61 73.12,56.2 72.16,56.2 72.16,55.88 | 72.16,55.88 72.16,55.25 72.8,55.25 72.8,55.88 72.16,55.88 | R29.1 67.4,72.07 T1.E
  Bottom 0.813: K24.15 13.43,62.23 24.86,50.8 IO8.10 | 29.94,50.8 35.02,45.72 | IO8.17 IO8.16 IO8.15 40.41,40.64 | K20.5 52.8,63.5 | 23.59,25.4 23.59,24.48 23.59,18.63 24.86,18.63 24.86,15.24 | C24.2 C23.2 | K4.3 31.21,26.67 | 15.76,27.86 15.76,29.21 5.17,29.21 IO11.4 IO11.3 | C30.2 C29.2 | K27.11 K25.6 | C20.- 108.26,47.2 | C22.2 C21.2 | C34.2 C33.2 106.14,33.02 | C31.2 C32.2 36.29,27.31 36.29,32.39 43.91,32.39 43.91,40.32 | C27.2 C28.2 69.94,69.75 IO1.8 | K20.1 52.8,58.42 52.8,62.86 61.05,62.86 61.05,64.45 PP1.3 | K25.25 K26.13 54.07,22.86 54.07,38.73 | K25.20 K27.4 62.96,5.08 LED1.K | K25.14 K27.7 | K26.5 K25.9 | 43.91,40.32 54.07,40.32 54.07,38.73 | K19.1 54.07,38.73 | IO9.P$14 105.5,65.41 | 106.14,32.39 106.14,33.02 | 106.14,33.02 106.14,35.56 | 40.41,40.64 40.41,40.32 43.91,40.32 | 28.67,26.67 v36.29,26.67 | 106.77,27.31 106.77,28.89 | v106.77,38.1 106.77,37.78 106.77,29.21 106.77,28.89 | 68.35,56.83 68.35,53.66 | K1.1 86.45,58.74 v86.45,41.59 | K14.1 106.77,28.89 | T4.E 68.04,55.25 | TL2-COM.1 40.41,40.64 | v110.27,80.52 110.27,80.53 109.94,80.53 | 120.74,38.73 120.74,33.97 119.15,33.97 119.15,40.32 120.74,40.32 120.74,38.73 | 119.47,40.32 119.47,34.61 120.11,34.61 K28.1 | K28.1 120.11,40 | K28.1 120.74,38.73
  Bottom 1.016: D6.A 126.46,73.03 117.57,73.03 116.3,74.3 116.3,80.52 v110.27,80.52 109.94,80.53 106.77,80.53 105.5,78.11 | 105.5,78.11 IO9.P$9 | 105.5,65.41 105.5,78.11
  Bottom 1.422: D6.A P43.1 D5.A
  Bottom 1.778: P44.1 106.77,37.78 | 61.05,64.45 61.05,65.09
GND2
  Top 0.813: C10.2 C11.2 103.91,20.42 103.91,22.22 104.86,23.18 109.67,23.18 109.63,23.21 K14.2
  Bottom 0.813: 109.67,24.75 K14.2 109.63,25.08 | 109.67,24.75 109.67,23.18 K15.2 | IO7.5 109.67,20.12 | 109.67,20.12 109.67,24.75 | 109.67,20.12 109.67,11.28 K16.6
GNDB2  (via drill 0.7)
  Top 0.61: IO5.10 147.09,48.26
  Top 0.813: B1.- 166.14,40.64 IO5.16 | 147.09,48.26 145.82,46.99 145.82,38.1 | 145.82,38.1 145.82,34.92 150.59,34.92 153.44,32.07 153.44,8.89 I04.4 150.9,6.67 144.55,6.67 v144.55,9.21 | K30.6 145.82,38.1
  Bottom 0.406: IO5.17 154.71,43.18
  Bottom 0.61: 149.63,48.26 IO5.10
  Bottom 0.813: B1.- 168.68,37.47 168.68,50.8 K10.6 | IO5.17 IO5.16 C9.2 C8.1 159.79,43.18 | 154.71,43.18 149.63,48.26 | CT2.2 138.83,10.48 140.11,9.21 v144.55,9.21 | C6.2 154.18,8.89 | 154.18,8.89 C7.2 154.18,12.06 155.35,12.06 155.35,13.97 | I04.4 154.18,8.89 | 155.35,13.97 155.35,16.51 C4.1 | 155.35,13.97 C5.2
GPA0
  Bottom 0.61: K10.7 IO5.21
  Bottom 0.813: IO5.21 K11.1 K10.7
GPA1
  Bottom 0.61: IO5.22 K10.9
  Bottom 0.813: IO5.22 K11.2 K10.9
GPA2
  Bottom 0.61: IO5.23 K10.11
  Bottom 0.813: IO5.23 K11.3 K10.11
GPA3
  Bottom 0.61: K10.13 IO5.24
  Bottom 0.813: IO5.24 K11.4 K10.13
GPA4
  Bottom 0.61: IO5.25 K10.15
  Bottom 0.813: IO5.25 K11.5 K10.15
GPA5
  Bottom 0.813: IO5.26 K11.6 K10.17
GPA6
  Bottom 0.813: IO5.27 K11.7 K10.19
GPA7
  Bottom 0.813: IO5.28 K11.8 K10.21
GPB0
  Bottom 0.61: IO5.1 149.63,71.12 | 150.9,69.85 164.87,69.85 K10.22
  Bottom 0.813: K12.1 IO5.1 | 149.63,71.12 150.9,69.85
GPB1
  Bottom 0.406: IO5.2 149.63,68.58
  Bottom 0.61: 150.9,67.31 164.87,67.31 K10.20
  Bottom 0.813: K12.2 IO5.2 | 149.63,68.58 150.9,67.31
GPB2
  Bottom 0.406: IO5.3 149.63,66.04
  Bottom 0.61: 150.9,64.77 164.87,64.77 K10.18
  Bottom 0.813: K12.3 IO5.3 | 149.63,66.04 150.9,64.77
GPB3
  Bottom 0.406: IO5.4 149.63,63.5
  Bottom 0.61: 150.9,62.23 164.87,62.23 K10.16
  Bottom 0.813: K12.4 IO5.4 | 149.63,63.5 150.9,62.23
GPB4
  Bottom 0.406: IO5.5 149.63,60.96
  Bottom 0.61: K10.14 164.87,59.69 150.9,59.69
  Bottom 0.813: K12.5 IO5.5 | 149.63,60.96 150.9,59.69
GPB5
  Bottom 0.406: IO5.6 149.63,58.42
  Bottom 0.61: K10.12 164.87,57.15 150.9,57.15
  Bottom 0.813: K12.6 IO5.6 | 149.63,58.42 150.9,57.15
GPB6
  Bottom 0.406: IO5.7 149.63,55.88
  Bottom 0.61: K10.10 164.87,54.61 150.9,54.61
  Bottom 0.813: K12.7 IO5.7 | 149.63,55.88 150.9,54.61
GPB7
  Bottom 0.406: IO5.8 149.63,53.34
  Bottom 0.61: K10.8 164.87,52.07 150.9,52.07
  Bottom 0.813: K12.8 IO5.8 | 149.63,53.34 150.9,52.07
INA1
  Top 0.61: IO3.1 16.6,65.41 8.35,65.41
  Top 0.813: 8.35,65.41 8.35,68.58 K5.2
INA2
  Top 0.61: IO3.2 17.87,64.14
  Top 0.813: 17.87,64.14 5.17,64.14 K5.3
IND12
  Top 0.61: IO3.12 19.14,70.48 17.24,68.58 13.43,68.58 12.16,67.31 K6.3
IND13
  Top 0.61: IO3.13 17.87,71.12 16.6,69.85 K6.2
IR-OUT
  Bottom 0.813: K7.1 K7.2 68.04,7.62 83.91,7.62 LED2.K
K24-1
  Bottom 0.61: K24.1 K37.3
  Bottom 0.813: K37B.3 K37.3
K24-2
  Bottom 0.61: K24.2 9.62,42.55 21.05,42.55
  Bottom 0.813: 21.05,42.55 K36.1
K24-3
  Bottom 0.61: K24.3 K37.2
  Bottom 0.813: K37B.2 K37.2
K24-4
  Bottom 0.61: K24.4 10.89,45.72 K36.2
K24-5
  Bottom 0.61: K24.5 K37.1
  Bottom 0.813: K37B.1 K37.1
K24-6
  Bottom 0.61: K24.6 10.89,48.26 K36.3
LED-A
  Top 0.813: LED-A2.A 56.83,29.62 LED-A1.A
  Bottom 0.61: R45.2 57.87,27.94 56.61,29.21
  Bottom 0.813: 56.61,29.21 LED-A1.A
LED-B
  Top 0.813: LED-B2.A 63.18,29.62 LED-B1.A
  Bottom 0.61: R46.2 61.69,27.94 62.96,29.21
  Bottom 0.813: 62.96,29.21 LED-B1.A
LED-C
  Top 0.813: LED-C2.A 69.53,29.62 LED-C1.A
  Bottom 0.61: R47.2 70.57,27.94 69.31,29.21
  Bottom 0.813: 69.31,29.21 LED-C1.A
LED-D
  Top 0.813: LED-D1.A 77.02,29.84 LED-D2.A
  Bottom 0.61: R48.2 76.92,27.94 75.66,29.21
  Bottom 0.813: 75.66,29.21 LED-D1.A
LED-PIN51
  Bottom 0.813: P51.1 58.51,32.7 R45.1
LED-PIN52
  Bottom 0.813: P52.1 61.05,32.7 R46.1
LED-PIN53
  Bottom 0.813: R47.1 73.75,29.84 73.75,31.43 P53.1
LED-PIN54
  Bottom 0.813: P54.1 R48.1
N$1
  Bottom 0.813: IO8.1 32.48,73.66 K18.1
N$2
  Top 0.813: IO8.2 31.21,71.12 31.21,76.2 29.94,76.2 K18.2
N$3
  Bottom 0.813: IO8.3 26.13,68.58 26.13,76.2 27.4,76.2 K18.3
N$4
  Bottom 0.813: K18.4 24.86,66.04 IO8.4
N$5
  Bottom 0.813: IO8.5 22.32,63.5 D4.C
N$6
  Bottom 0.813: D4.A K18.5
N$7
  Bottom 0.813: D3.C 19.78,63.5 22.32,60.96 IO8.6
N$8
  Bottom 0.813: D3.A K18.6
N$9
  Bottom 0.813: IO8.7 22.32,58.42 17.24,63.5 D2.C
N$10
  Bottom 0.813: D2.A K18.7
N$11
  Bottom 0.813: D1.C 14.7,63.5 22.32,55.88 IO8.8
N$12
  Bottom 0.813: D1.A K18.8
N$13
  Bottom 0.813: K25.23 K26.12
N$14
  Top 0.813: R41.2 89.63,54.29 P47.1
N$15
  Top 0.813: K29.9 K31.1
N$17
  Bottom 0.813: K25.21 K26.11
N$18
  Bottom 0.61: P16.1 164.03,16.51
  Bottom 0.813: 164.03,16.51 D9.1 D8.1 | CT1.2 158.52,21.59 I04.8 P16.1
N$19
  Bottom 0.813: K25.19 K26.10
N$20
  Top 0.813: K8.1 I04.6 155.98,11.43 155.98,20.96 R8.2
N$21
  Bottom 0.813: K25.13 K26.7
N$22
  Top 0.61: K20.11 48.99,69.85 45.18,69.85
  Top 0.813: 45.18,69.85 45.18,55.88 IO8.21
N$23
  Bottom 0.61: K20.12 48.99,69.85 48.99,59.69 46.45,59.69
  Bottom 0.813: IO8.22 37.56,58.42 38.83,59.69 46.45,59.69
N$24
  Top 0.61: K20.13 48.99,72.39 43.91,72.39 43.91,70.17 42,70.17 40.73,68.9
  Top 0.813: 40.73,68.9 40.73,60.96 IO8.23
N$25
  Top 0.813: IO8.24 35.02,63.5 33.75,64.77 33.75,75.56 43.91,75.56 43.91,73.66 K20.14
N$26
  Bottom 0.813: K25.7 K26.4
N$27
  Top 0.813: K29.11 K31.3
N$28
  Bottom 0.813: IO8.25 38.83,66.04 38.83,62.23 40.1,60.96 K20.4
N$29
  Top 0.813: K8.2 I04.5 154.71,8.89 154.71,26.35 R9.2
N$30
  Bottom 0.813: IO8.26 38.83,68.58 40.1,67.31 40.1,64.77 41.37,63.5 K20.6
N$31
  Top 0.61: 124.87,37.78 125.5,37.78 | 126.14,37.78 125.5,37.78 | 125.5,37.78 125.5,38.42 | 125.5,37.78 125.5,37.15
N$32
  Top 0.813: K30.9 140.74,30.48 142.65,32.39 K32.1
N$33
  Bottom 0.813: IO8.27 P36.1 43.27,71.12 43.27,81.91 R27.1
N$34
  Bottom 0.61: R27.2 P35.1 R28.1
  Bottom 0.813: 59.78,81.91 P35.1
N$35
  Bottom 0.61: R26.1 62.32,78.11 T1.C
N$36
  Bottom 0.61: R26.2 55.97,78.11
  Bottom 0.813: K20.16 47.72,78.11 55.97,78.11 57.24,78.11
N$37  (via drill 0.7)
  Top 0.61: 94.07,16.51 99.15,16.51
  Top 0.813: v107.41,16.51 99.15,16.51 | 94.07,16.51 92.8,16.51 R18.2
  Bottom 0.406: 107.41,17.15 v107.41,16.51 | 107.41,8.86 K16.1
  Bottom 0.61: IO7.6 105.5,19.05 107.41,17.15
  Bottom 0.813: v107.41,16.51 107.41,8.86
N$38
  Top 0.813: K30.11 140.74,25.4 142.65,27.31 K32.3
N$40
  Bottom 0.813: I04.3 147.41,11.43 P17.1 147.41,6.35 R11.1
N$41
  Bottom 0.406: 96.61,11.43 96.61,11.33
  Bottom 0.61: K16.8 96.61,11.33 | K13.1 95.98,20.32 96.61,19.69 96.61,13.97
  Bottom 0.813: 96.61,11.43 96.61,13.97
N$43
  Top 0.813: R15.1 46.45,4.13 LED3.A
N$47
  Bottom 0.813: K19.9 P32/G.1
N$48
  Bottom 0.813: K19.7 P32/E.1
N$49
  Bottom 0.813: K19.5 P32/C.1
N$50
  Bottom 0.813: K19.3 P32/A.1
N$51
  Top 0.61: R41.1 95.97,52.39 92.48,52.39 P48.1
  Top 0.813: R42.2 R41.1
N$58
  Bottom 0.813: P32/B.1 55.65,44.45 61.05,44.45 K19.4
N$59
  Bottom 0.813: K19.6 63.59,46.36 58.19,46.36 P32/D.1
N$61
  Top 0.813: Q1.1 75.24,55.59 C1.1 75.34,60.96 R1.1 75.34,65.09 IO1.11
N$62
  Top 0.61: IO1.10 72.48,61.59 | R1.2 72.48,61.59 | 72.48,61.59 R2.2
N$64
  Top 0.813: 69.75,61.28 C3.1 | C3.1 69.73,61.28 R2.1 | Q1.2 69.73,55.59 C3.1
N$72
  Bottom 0.813: P37.1 IO8.28
N$79
  Top 0.406: T2.2 36.6,7.62 | R12.2
  Top 0.813: 36.6,7.62 36.6,6.67 R12.2 | R12.2 R14.2
N$81
  Top 0.813: R15.2 38.19,4.13 T2.1
N$82
  Bottom 0.813: K25.11 K26.6
N$83
  Top 0.813: R12.1 P19.1
N$84
  Bottom 0.813: K25.15 K26.8
N$85
  Bottom 0.813: K25.17 K26.9
N$86
  Bottom 0.813: K19.10 73.75,41.28 P32/H.1
N$87
  Bottom 0.813: K27.10 K25.8
N$88
  Bottom 0.813: K25.10 K27.9
N$89
  Bottom 0.813: K20.8 P40.1
N$90
  Bottom 0.813: K27.6 K25.16
N$91
  Bottom 0.813: K27.8 K25.12
N$92
  Bottom 0.813: K27.2 K25.24
N$93
  Bottom 0.813: K27.3 K25.22
N$94
  Bottom 0.813: K27.1 K25.26
N$95
  Bottom 0.813: K27.5 K25.18
N$96
  Bottom 0.813: K20.10 P41.1
N$97
  Bottom 0.813: K20.9 55.34,68.58 P39.1
N$98
  Bottom 0.61: 54.7,66.04 P38.1
  Bottom 0.813: K20.7 54.7,66.04
N$103
  Bottom 0.813: K19.8 66.13,46.99 P32/F.1
N$105
  Top 0.61: 102.33,6.32 K16.2
  Top 0.813: 102.33,6.32 102.33,3.18 92.8,3.18 R17.2
  Bottom 0.61: IO7.7 104.23,18.41
  Bottom 0.813: 104.23,18.41 104.23,13.34 104.87,12.7 104.87,8.89 104.84,8.89 K16.2
N$108
  Bottom 0.813: K16.3 113.76,8.83 K15.1
N$109
  Bottom 1.27: K16.SH1 99.34,5.03 K16.SH2 112.89,5.03 K16.SH3
N$111
  Top 0.813: R3.1 80.1,61.59 K1.3
  Bottom 0.813: K1.2 K1.3 77.56,58.74 IO1.12
N$112
  Bottom 0.813: T4.C 57.56,60.33 P25.1 D10.A
N$113
  Top 0.813: T4.B 65.5,57.78 | 65.5,57.78 R20.2 | 65.5,57.78 R21.2
N$114
  Top 0.813: P24.1 69.31,50.8 65.5,54.29 R20.1
N$115
  Top 0.813: IO8.19 P31.1
N$117
  Bottom 0.406: R10.1 164.87,13.97
  Bottom 0.813: 155.88,6.35 164.87,6.35 164.87,13.97 | 155.88,6.35 C6.1 C7.1 | R11.2 155.88,6.35 | R19.2 167.73,29.21 | 167.73,29.21 167.73,15.24 169.64,15.24 P18.1 169.64,13.97 R10.1 | 167.73,29.21 160.63,29.21 D8.2
N$118
  Bottom 0.813: IO9.P$10 100.74,75.56 K22.4
N$119
  Bottom 0.813: R7.2 81.37,5.72 LED2.A
N$120
  Bottom 0.813: LED1.A R6.2
N$121
  Bottom 0.813: P14.1 R6.1
N$122
  Top 0.813: 21.68,27.94 21.68,22.22
N$123
  Top 0.813: 22.95,22.22 22.95,27.94
N$124
  Top 0.813: 24.22,27.94 24.22,22.22
N$125
  Top 0.813: 25.49,27.94 25.49,22.22
N$126
  Top 0.813: 26.76,27.94 26.76,22.22
N$127
  Top 0.813: 28.03,27.94 28.03,22.22
N$128
  Top 0.813: 29.3,27.94 29.3,22.22
N$129
  Top 0.813: 21.68,20.32 21.68,14.6
N$130
  Top 0.813: 22.95,20.32 22.95,14.6
N$131
  Top 0.813: 24.22,20.32 24.22,14.6
N$132
  Top 0.813: 25.49,20.32 25.49,14.6
N$133
  Top 0.813: 26.76,20.32 26.76,14.6
N$134
  Top 0.813: 28.03,20.32 28.03,14.6
N$135
  Top 0.813: 29.3,20.32 29.3,14.6
N$136
  Bottom 0.813: IO9.P$11 101.06,73.03 96.61,68.58 96.61,66.36 K22.3
N$140
  Top 0.813: IO5.20 161.7,50.8 161.7,73.66 P22.1
N$141
  Top 0.813: P23.1 153.44,73.66 153.44,48.26 IO5.19
N$145
  Top 0.813: P20.1 K10.3
N$146
  Top 0.813: K10.4 168.68,48.26 168.68,73.03 163.6,73.03 P21.1
N$151
  Bottom 0.813: K22.2 98.2,63.82 98.2,67.94 100.74,70.48 IO9.P$12
N$154
  Bottom 0.813: IO9.P$13 101.06,67.94 100.1,66.99 100.1,61.28 K22.1
N$157
  Top 0.813: R43.2 91.53,57.78 91.53,62.86 P49.1
N$160
  Top 0.61: R43.1 94.7,55.88 89.63,55.88 P50.1
  Top 0.813: R44.2 R43.1
N$164
  Top 0.813: 20.41,22.22 20.41,27.94
N$181
  Bottom 0.61: R28.2 T1.B R29.2
N$183
  Top 0.813: R35.2 R34.1 108.04,54.29 STAB1.1
N$1123
  Top 0.813: 20.41,20.32 20.41,14.6
OUTA3
  Top 0.61: IO3.3 19.14,67.94 19.78,68.58
  Top 0.813: 19.78,68.58 26.13,68.58 26.13,77.47 12.79,77.47 12.79,74.3 5.17,74.3 K5.1
OUTD11
  Top 0.61: 20.41,74.93 IO3.11
  Top 0.813: K6.1 14.7,72.39 14.7,74.93 20.41,74.93
PWM0
  Bottom 0.305: IO2.6 34.38,23.84
  Bottom 0.61: 34.38,23.84 PWM0.1
PWM1
  Bottom 0.305: IO2.7 32.48,23.19
  Bottom 0.406: 32.48,23.19 32.48,21.59
  Bottom 0.813: 32.48,21.59 PWM1.1
PWM2
  Bottom 0.305: IO2.8 29.3,22.53
  Bottom 0.406: 29.3,22.53 33.11,18.73 33.11,14.92 29.62,14.92
  Bottom 0.61: 2,13.97 2,62.23 K24.16
  Bottom 0.813: 2,13.97 9.62,13.97 12.16,12.06 19.14,12.06 19.14,7.94 29.62,7.94 29.62,14.92
PWM3
  Bottom 0.305: IO2.9 26.5,21.91 28.67,21.91
  Bottom 0.406: 28.67,21.91 32.16,18.41 32.16,16.19 28.03,16.19 28.03,15.56
  Bottom 0.61: 3.27,15.24 3.27,59.69 K24.14
  Bottom 0.813: 3.27,15.24 11.52,15.24 11.52,14.6 13.11,13.34 20.41,13.34 20.41,9.21 28.03,9.21 28.03,15.56
PWM4
  Bottom 0.305: 30.31,17.82 30.3,17.83 30.34,17.83 30.34,17.8 30.32,17.8 | 30.31,17.82 | IO2.10 26.5,21.21 28.22,21.21
  Bottom 0.406: 28.22,21.21 30.3,19.13 30.3,17.83
  Bottom 0.813: 30.32,17.78 31.21,17.78 31.21,17.15 30.25,17.15 30.25,17.78 30.32,17.78 | 30.32,17.8 30.32,17.78
PWM5
  Bottom 0.305: IO2.11 27.64,20.58
  Bottom 0.406: 27.64,20.58 28.46,19.76 28.46,17.98
  Bottom 0.813: 28.46,17.78 27.4,17.78 27.4,17.15 28.98,17.15 28.98,17.78 28.67,17.78 28.46,17.78 | 28.46,17.98 28.46,17.78
PWM8
  Bottom 0.406: IO2.15 20.67,17.46 16.28,17.46
  Bottom 0.813: PWM8.1 16.28,17.46
PWM9
  Bottom 0.406: IO2.16 14.38,19.28
  Bottom 0.813: 14.38,19.28 14.38,19.37 | 14.38,19.37 PWM9.1 | 14.38,19.37 18.82,19.37
PWM11
  Bottom 0.305: IO2.18 22.32,20.59
  Bottom 0.61: 22.32,19.69 22.32,20.32
  Bottom 0.813: 22.32,20.59 22.32,19.69 22.32,17.78 21.05,16.51 17.24,16.51 17.24,15.24 PWM11.1
PWM12
  Bottom 0.406: IO2.19 12.75,21.23 8.98,17.15
  Bottom 0.813: 8.98,17.15 PWM12.1
PWM13
  Bottom 0.406: IO2.20 11.82,21.88
  Bottom 0.813: PWM13.1 9.62,19.37 11.82,21.88
PWM14
  Bottom 0.406: IO2.21 14.38,22.53 14.38,22.86
  Bottom 0.813: PWM14.1 14.38,22.86
PWM15
  Bottom 0.406: IO2.22 17.87,23.19 17.87,24.13
  Bottom 0.813: 17.87,24.13 15.97,26.03 PWM15.1
PWM-EXTCLK
  Bottom 0.305: IO2.25 22.05,25.13
  Bottom 0.406: 22.05,25.13 25.49,28.57
  Bottom 0.813: 25.49,28.57 28.67,28.57 K4.2
PWR+
  Top 0.813: 123.6,40.32 122.01,40.32 122.01,33.97 123.6,33.97 123.6,40.32 | 123.6,40.32 122.96,39.69 122.96,38.73 | 122.96,38.73 122.96,34.29 122.65,34.29 K28.2 | K28.2 122.65,40 | K28.2 122.96,38.73
  Bottom 0.305: 122.79,38.73 K28.2
  Bottom 0.813: 122.96,40.32 123.6,40.32 123.6,33.97 122.01,33.97 122.01,40.32 122.33,40.32 | 122.96,40.32 122.65,40.32 | 122.65,40.32 122.33,40.32 | 122.79,40.64 122.65,40.64 122.65,40.32 | 122.33,40.32 122.33,34.61 122.96,34.61 122.96,40.32
  Bottom 1.422: F2.2 F1.2 122.79,40.64 122.79,38.73
RPI-G1
  Top 0.813: IO6.2 40.73,26.03 42.64,27.94 P27.1
  Bottom 0.813: P27.1 43.91,30.48 R24.1
RPI-G2
  Top 0.813: IO6.3 39.46,29.84 P28.1
RTC-INT
  Top 0.813: K29.7 P46.1
RTC-INT-B2  (via drill 0.7)
  Top 0.813: I04.7 164.74,13.97 164.74,5.08 142.65,5.08 142.65,9.21 140.43,9.21 140.43,12.38 142.33,14.29 142.33,15.56 140.11,17.78 v140.11,22.22
  Bottom 0.813: I04.7 R10.2 | v140.11,22.22 140.11,22.86 142.01,24.13 142.01,35.56 K30.7
RTC-P1
  Bottom 0.406: 143.92,16.19 143.92,16.51
  Bottom 0.813: 148.36,16.51 I04.1 C4.2 | 148.36,16.51 148.05,16.51 | 148.05,16.51 147.73,16.51 CT1.1A | 143.92,16.51 143.92,18.42 | 143.92,18.42 PCT1.1 | Q2.2 145.82,16.19 | CT2.1A 143.92,18.42 | PCT2.1 145.82,16.19 | 145.82,16.19 143.92,16.19 | Q2.2 148.05,16.51 | Q2.2 148.36,16.19 148.36,16.51
  Bottom 1.778: 148.36,15.88 148.36,16.51 148.36,19.05 147.41,19.05 147.41,15.88 148.36,15.88
RTC-P2
  Bottom 0.813: C5.1 I04.2 148.68,13.97 | 148.68,13.97 147.41,13.97 147.41,12.7 148.68,12.7 | 148.68,12.7 149,12.7 149,13.65 Q2.1 | 148.68,12.7 148.68,13.97
SCL3  (via drill 0.7)
  Top 0.61: v105.5,29.21 v86.13,29.21 | IO10.2 82.64,34.29
  Top 0.813: v86.13,29.21 82.64,32.39 82.64,34.29
  Bottom 0.61: IO7.3 v105.5,29.21
  Bottom 0.813: K25.5 K26.3 80.74,29.21 v86.13,29.21
SCL3-VOLIT
  Top 0.813: K29.2 K33.1
SCL3-VOLIT-B2
  Top 0.61: 146.46,49.53 150.27,49.53 | 153.44,44.45 157.89,44.45
  Top 0.813: 150.27,49.53 150.9,49.53 150.9,44.45 153.44,44.45 | 157.89,44.45 159.16,43.18 166.14,43.18 K10.2 | 146.46,49.53 145.82,49.53 144.55,48.26 K30.2
  Bottom 0.813: K34.1 141.06,56.83 141.06,48.26 K30.2
SCL5  (via drill 0.7)
  Top 0.61: IO10.7 82.64,43.18
  Top 0.813: v40.1,35.56 54.07,35.56 54.07,36.83 76.29,36.83 v76.29,41.91 | R39.2 v82.64,49.53 82.64,43.18 K35.3 K29.4 | K24.11 26.13,57.15 26.13,45.72 IO8.12
  Bottom 0.406: IO2.26 19.39,25.78 17.24,27.94 | IO11.6 17.24,33.66
  Bottom 0.61: 17.24,33.66 17.24,27.94
  Bottom 0.813: IO11.6 22.95,33.66 24.86,35.56 24.86,45.72 IO8.12 30.57,45.72 32.48,43.81 32.48,37.47 36.29,37.47 36.29,35.56 v40.1,35.56 | v76.29,41.91 76.29,49.53 v82.64,49.53
SCL5B2
  Top 0.813: IO5.12 153.44,43.18 153.44,36.83 155.98,34.29 157.57,34.29 R8.1
  Bottom 0.813: K30.4 IO5.12
SDA3  (via drill 0.7)
  Top 0.61: IO10.3 83.91,34.29
  Top 0.813: 83.91,34.29 v87.72,30.8
  Bottom 0.61: IO7.2 104.23,22.86
  Bottom 0.813: K25.3 K26.2 83.28,27.31 87.72,27.31 | 87.72,27.31 88.99,27.31 88.99,22.86 104.23,22.86 | v87.72,30.8 87.72,27.31
SDA3-VOLIT
  Top 0.813: K29.1 K33.2
SDA3-VOLIT-B2
  Top 0.61: 157.89,46.99 152.17,46.99 | 152.17,52.07 146.46,52.07
  Top 0.813: 157.89,46.99 159.16,45.72 K10.1 | 152.17,46.99 152.17,52.07 | 146.46,52.07 145.82,52.07 144.55,50.8 K30.1 K34.2
SDA5  (via drill 0.7)
  Top 0.61: 26.76,59.69 31.21,59.69 | 85.82,39.37 83.91,39.37 | IO10.6 83.91,39.37 | 83.91,39.37 80.74,39.37
  Top 0.813: v18.51,31.11 IO11.5 | v40.1,33.66 55.97,33.66 55.97,35.24 78.2,35.24 78.2,39.37 | 78.2,39.37 v78.2,41.91 | v84.55,45.08 84.55,52.7 R40.2 | K24.13 26.76,59.69 | 31.21,59.69 31.21,43.18 IO8.13 | 78.2,39.37 80.74,39.37 | 85.82,39.37 87.09,39.37 88.36,40.64 K35.2 K29.5
  Bottom 0.406: IO2.27 20.01,26.44 18.51,27.94
  Bottom 0.61: 27.4,35.56 27.4,31.11
  Bottom 0.813: 18.51,27.94 v18.51,31.11 27.4,31.11 | v78.2,41.91 78.2,45.08 v84.55,45.08 | v40.1,33.66 33.11,33.66 33.11,36.19 31.21,36.19 31.21,42.55 30.57,43.18 IO8.13 26.13,43.18 26.13,38.73 27.4,37.47 27.4,35.56
SDA5B2
  Top 0.813: IO5.13 151.86,40.64 151.86,36.19 154.71,33.34 154.71,28.25 R9.1
  Bottom 0.813: K30.5 IO5.13
SPOL-FREQ
  Top 0.61: 35.65,80.01 32.48,76.83
  Top 0.813: P1.1 35.65,80.01 | 32.48,76.83 32.48,36.83 26.13,36.83 K4.1
  Bottom 0.813: P1.1 69.31,82.23 K2.2 K2.4 K2.6 K2.8 K2.10 K2.12 K2.14 K2.16 K2.18 K2.20 K2.22
TL1-NO
  Bottom 0.813: R49.1 | P55.1 31.21,5.4 R49.1 | TL1-NO.1 21.36,2.86 R49.1
TL2-NO  (via drill 0.7)
  Top 0.813: v46.13,37.15 39.46,37.15 39.46,40.32 45.49,40.32 TL2-NO.1
  Bottom 0.813: TL2-NO.1 P56.1 | R50.1 v46.13,37.15
VDD2
  Top 0.813: K13.6 97.88,8.83 | 97.88,8.83 K16.5 | R17.1 R18.1 92.8,8.83 97.88,8.83 | C10.1 C11.1 K13.2
  Bottom 0.61: IO7.8 102.96,17.78
  Bottom 0.813: K13.6 K13.4 | 102.96,17.78 K13.4 | K13.4 K13.2
VDD-2
  Top 0.305: C12.1 47.08,22.86
  Top 0.61: R22.1 45.81,13.97 45.81,19.13 42,19.13 IO6.8
  Top 0.813: 45.81,19.13 46.66,19.13 C13.1 C12.1 | 47.08,22.86 K17.2 | R23.1 R22.1
VOLIT2-B1
  Top 0.813: K31.2 K29.10
VOLIT2-B2
  Top 0.813: K30.10 140.74,27.94 142.65,29.84 K32.2
VREF  (via drill 0.7)
  Top 0.813: v110.9,52.39 R34.2
  Bottom 0.813: IO9.P$15 105.5,62.86 105.5,57.78 | K21.8 124.55,60.33 124.55,52.39 v110.9,52.39 110.9,57.78 105.5,57.78 | STAB1.3 105.5,56.52 | 105.5,57.78 105.5,56.52 | 105.5,56.52 R36.1
(copper drawn outside any net)
  shapes: Top circle x3

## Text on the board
Top: RPi-EXP. | D2-v_12 | RPi-EXP. | D1-v_12
Bottom: D2-v_12 | + | D1-v_12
